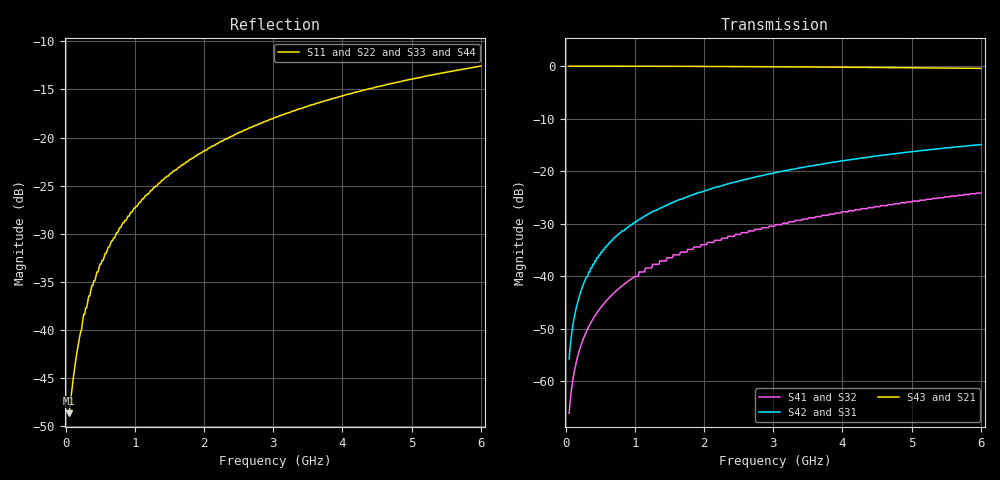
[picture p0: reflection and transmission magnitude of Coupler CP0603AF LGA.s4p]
!	AVX THIN FILM OPERATION
!	CP0603 HIGH DIRECTIVITY COUPLERS
!	P/N CP0603AxxxxFLTR
!	Network	Analyzer HP8720ES.07.64:Feb23,2000 Serial No.US39172382
!	Hewlett-Packard
!	24 July 2003	02:45:57
# MHZ S MA R 50
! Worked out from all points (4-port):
!   400 points, 50 MHz to 6 GHz, reference 50 ohm
!   strongest paths, dB at 50 MHz, 1.541 GHz, 3.032 GHz, 4.524 GHz, 6 GHz:
!     S43: 0.0, -0.1, -0.1, -0.3, -0.4
!     S21: 0.0, -0.1, -0.1, -0.3, -0.4
!     S42: -55.7, -26.0, -20.3, -17.1, -14.9
!     S31: -55.7, -26.0, -20.3, -17.1, -14.9
!     S41: -66.1, -36.5, -30.2, -26.7, -24.2
!     S32: -66.1, -36.5, -30.2, -26.7, -24.2
!   lowest |S11| = -48.7 dB at 50 MHz (marker M1), VSWR 1.01, Z = 50.3 - j0.217 ohm
!   |S11| at or under -10 dB: start of sweep to end of sweep
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50  0.003682 -36.0  0.997 -0.2  0.001639 89.8  0.0004976 89.5
    0.997 -0.2  0.003682 -36.0  0.0004976 89.5  0.001639 89.8
    0.001639 89.8  0.0004976 89.5  0.003682 -36.0  0.997 -0.2
    0.0004976 89.5  0.001639 89.8  0.997 -0.2  0.003682 -36.0
154.386  0.007281 -66.4  0.997 -0.6  0.005059 89.3  0.001537 88.1
         0.997 -0.6  0.007281 -66.4  0.001537 88.1  0.005059 89.3
         0.005059 89.3  0.001537 88.1  0.007281 -66.4  0.997 -0.6
         0.001537 88.1  0.005059 89.3  0.997 -0.6  0.007281 -66.4
363.158  0.016 -80.7  0.997 -1.4  0.012 88.3  0.003615 85.6
         0.997 -1.4  0.016 -80.7  0.003615 85.6  0.012 88.3
         0.012 88.3  0.003615 85.6  0.016 -80.7  0.997 -1.4
         0.003615 85.6  0.012 88.3  0.997 -1.4  0.016 -80.7
691.228  0.03 -87.2  0.996 -2.6  0.023 86.9  0.006885 81.7
         0.996 -2.6  0.03 -87.2  0.006885 81.7  0.023 86.9
         0.023 86.9  0.006885 81.7  0.03 -87.2  0.996 -2.6
         0.006885 81.7  0.023 86.9  0.996 -2.6  0.03 -87.2
1153.509  0.05 -91.4  0.995 -4.3  0.038 84.8  0.012 76.2
          0.995 -4.3  0.05 -91.4  0.012 76.2  0.038 84.8
          0.038 84.8  0.012 76.2  0.05 -91.4  0.995 -4.3
          0.012 76.2  0.038 84.8  0.995 -4.3  0.05 -91.4
2957.895  0.124 -100.8  0.984 -10.9  0.095 77.0  0.03 55.2
          0.984 -10.9  0.124 -100.8  0.03 55.2  0.095 77.0
          0.095 77.0  0.03 55.2  0.124 -100.8  0.984 -10.9
          0.03 55.2  0.095 77.0  0.984 -10.9  0.124 -100.8
6000  0.235 -112.9  0.95 -21.4  0.179 64.9  0.062 22.8
      0.95 -21.4  0.235 -112.9  0.062 22.8  0.179 64.9
      0.179 64.9  0.062 22.8  0.235 -112.9  0.95 -21.4
      0.062 22.8  0.179 64.9  0.95 -21.4  0.235 -112.9
